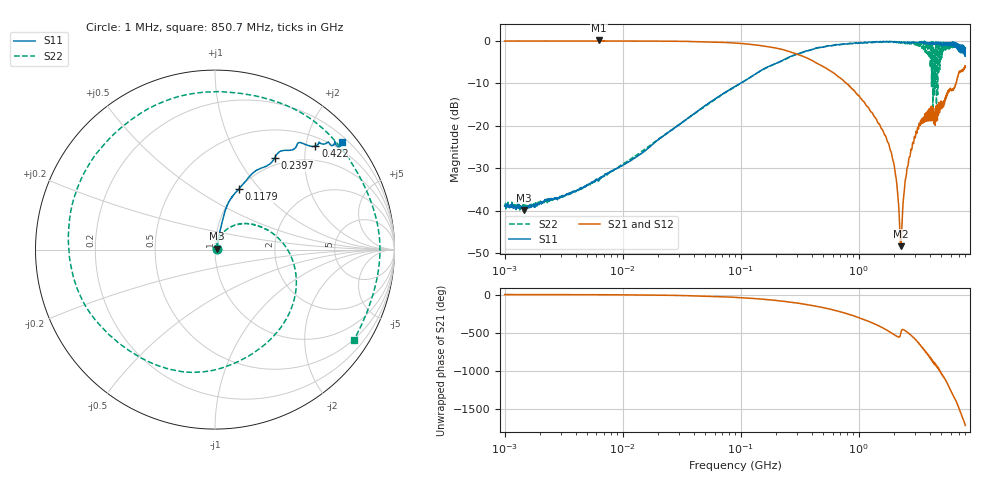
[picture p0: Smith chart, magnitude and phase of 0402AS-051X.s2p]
!s-Parameter Generated by FASTRON Sdn. Bhd.
!FASTRON P/N : 0402AS-051X
!Keysight Technologies: E5071C_MY46733604_B.14.02
!Date: Mon Dec 01 10:47:28 2025
!Version  :Rev00  Mon Dec 01 10:47:28 2025
!Data & Calibration Information:
!Freq  S11:SOLT2(ON)  S21:SOLT2(ON)  S12:SOLT2(ON)  S22:SOLT2(ON)
!PortZ  Port1:50+j0  Port2:50+j0
!When reading reference impedance value at option line is always used.
! Remarks : This data is being provided solely for informational purposes.
# Hz S dB R 50
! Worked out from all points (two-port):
!   1601 points, 1 MHz to 8 GHz, reference 50 ohm
!   highest |S21| = 0.03 dB at 6.301 MHz (marker M1); lowest = -48.3 dB at 2.267 GHz (marker M2)
!   |S21| within 3 dB of the highest: start of sweep to 283.8 MHz
!   lowest |S11| = -39.8 dB at 1.468 MHz (marker M3), VSWR 1.02, Z = 50.9 + j0.459 ohm
!   |S11| at or under -10 dB: start of sweep to 100 MHz
!   |S22| runs from -39.8 to -0.1 dB; largest |S21 - S12| = 0.016
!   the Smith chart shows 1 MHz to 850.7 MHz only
!   S11 on the Smith chart (normalised r, x): 1 MHz: 1.02, +0.01; 117.9 MHz: 1.00, +0.78; 239.7 MHz: 0.89, +1.45; 422 MHz: 0.67, +2.19; 850.7 MHz: 0.31, +2.69
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1000000  -38.90 22.4  -0.10 -0.5  -0.09 -0.4  -38.60 19.4
1468277  -39.80 26.1  -0.10 -0.7  -0.10 -0.6  -38.60 18.9
4479405  -34.50 54.4  -0.10 -1.9  -0.10 -1.9  -34.80 54.9
6301378  -32.40 64.8  0.03 -2.8  -0.07 -3.2  -32.10 58.9
2.00676e7  -23.30 74.5  -0.13 -8.6  -0.13 -8.5  -23.20 68.4
8.994653e7  -10.80 73.2  -0.57 -37.0  -0.56 -36.9  -10.80 25.6
1.178514e8  -8.81 68.5  -0.84 -47.9  -0.83 -47.9  -8.79 9.2
2.396863e8  -4.29 57.0  -2.30 -92.0  -2.29 -92.0  -4.38 -65.2
4.006501e8  -2.15 47.8  -4.65 -144.0  -4.64 -144.0  -2.07 -157.0
4.220185e8  -1.90 45.9  -5.01 -150.0  -4.99 -150.0  -1.91 -168.0
6.257563e8  -1.01 41.6  -7.79 153.0  -7.78 153.0  -1.10 82.5
8.506618e8  -0.65 40.4  -11.00 94.6  -10.90 94.5  -0.70 -33.2
1.1258e9  -0.37 43.5  -14.70 27.9  -14.70 27.8  -0.56 -172.0
1.334081e9  -0.29 49.1  -17.60 -19.3  -17.60 -19.4  -0.43 87.4
1.542898e9  -0.27 55.6  -20.50 -64.9  -20.50 -65.0  -0.28 -11.0
1.7949e9  -0.21 62.5  -24.30 -121.0  -24.30 -121.0  -0.38 -133.0
2.061212e9  -0.39 68.7  -32.00 -177.0  -32.00 -177.0  -0.35 99.7
2.266813e9  -0.45 72.3  -48.30 -148.0  -48.60 -148.0  -0.54 -3.2
2.618947e9  -0.46 81.8  -29.20 -141.0  -29.20 -141.0  -0.33 -175.0
2.985754e9  -0.41 92.3  -22.80 137.0  -22.70 136.0  -0.68 1.7
3.345355e9  -0.47 101.0  -18.70 50.6  -18.60 50.3  -1.49 -175.0
8e9  -1.69 -111.0  -6.23 88.2  -6.25 87.8  -3.31 124.0
